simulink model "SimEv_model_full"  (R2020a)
settings: Solver=VariableStepAuto  StartTime=0.0  StopTime=20  RelTol=1e-3
undefined symbols (not defined in the file): m, n

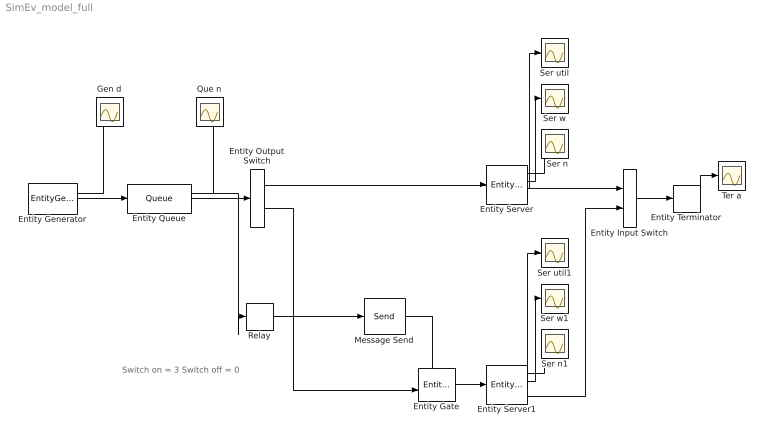
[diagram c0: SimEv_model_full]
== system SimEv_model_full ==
  note: Switch on = 3 Switch off = 0
  Entity Input Switch : EntityInputSwitch  InputPortMessageModes=m,m  OutputPortMessageModes=m
  Entity Output Switch : EntityOutputSwitch  InputPortMessageModes=m  OutputPortMessageModes=m,m  SwitchAttributeName=Attribute1
  Entity Gate : EntityGate  InputPortMessageModes=m,m  OutputPortMessageModes=m
  Entity Generator : EntityGenerator  OutputPortMessageModes=n,m  IntergenerationTimeAction=|  NumberEntitiesDeparted=on  EntityType=Structured  EntityTypeName=Entity
      | dt = rand(1,1);
      | persistent rngInit;
      | if isempty(rngInit)
      |     seed = 12345;
      |     rng(seed);
      |     rngInit = true;
      | end
      | 
      | % Pattern: Exponential distribution
      | mu = 1;
      | dt = -mu * log(1 - rand());
  Entity Queue : Queue  InputPortMessageModes=m  OutputPortMessageModes=n,m  NumberEntitiesInBlock=on
  Entity Server : EntityServer  InputPortMessageModes=m  OutputPortMessageModes=n,n,n,m  Capacity=1  ServiceTimeValue=2  ServiceTimeAction=dt = 2*rand(1,1);  NumberEntitiesInBlock=on  AverageWait=on  Utilization=on
  Entity Server1 : EntityServer  InputPortMessageModes=m  OutputPortMessageModes=n,n,n,m  Capacity=1  ServiceTimeValue=0.5  ServiceTimeAction=dt = 2*rand(1,1);  NumberEntitiesInBlock=on  AverageWait=on  Utilization=on
  Entity Terminator : EntityTerminator  InputPortMessageModes=m  NumberEntitiesArrived=on
  Gen d : Scope
  Message Send : Send  OutputPortMessageModes=m
  Que n : Scope
  Relay : Relay  OnSwitchValue=3  OffSwitchValue=0
  Ser n : Scope
  Ser n1 : Scope
  Ser util : Scope
  Ser util1 : Scope
  Ser w : Scope
  Ser w1 : Scope
  Ter a : Scope
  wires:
  Entity Generator/2 -> Entity Queue/1
  Entity Server/4 -> Entity Input Switch/1
  Entity Queue/2 -> Entity Output Switch/1
  Entity Generator/1 -> Gen d/1
  Entity Queue/1 -> Relay/1, Que n/1
  Entity Server/2 -> Ser w/1
  Entity Server/3 -> Ser util/1
  Entity Server/1 -> Ser n/1
  Entity Terminator/1 -> Ter a/1
  Entity Server1/1 -> Ser n1/1
  Entity Server1/3 -> Ser util1/1
  Entity Server1/2 -> Ser w1/1
  Entity Output Switch/1 -> Entity Server/1
  Entity Server1/4 -> Entity Input Switch/2
  Entity Input Switch/1 -> Entity Terminator/1
  Entity Gate/1 -> Entity Server1/1
  Entity Output Switch/2 -> Entity Gate/2
  Relay/1 -> Message Send/1
  Message Send/1 -> Entity Gate/1
